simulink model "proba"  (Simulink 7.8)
settings: Solver=ode45  StartTime=0.0  StopTime=0.06  RelTol=1e-3
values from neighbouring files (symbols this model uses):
  alfa = 5*10e-3/6    (= 0.00833333333333)    [parametri.m]
  C = 3*C    (= 0.0039788735773)    [parametri.m]
  L = 7.64e-3    (= 0.00764)    [parametri.m]
  Lm = (9.3e-3)/W    (= 2.96028194151e-05)    [parametri.m]
  Rl = 1    [parametri.m]
  Rm = 1.6e-3    (= 0.0016)    [parametri.m]
libraries: powerlib x15, powerlib_extras x1

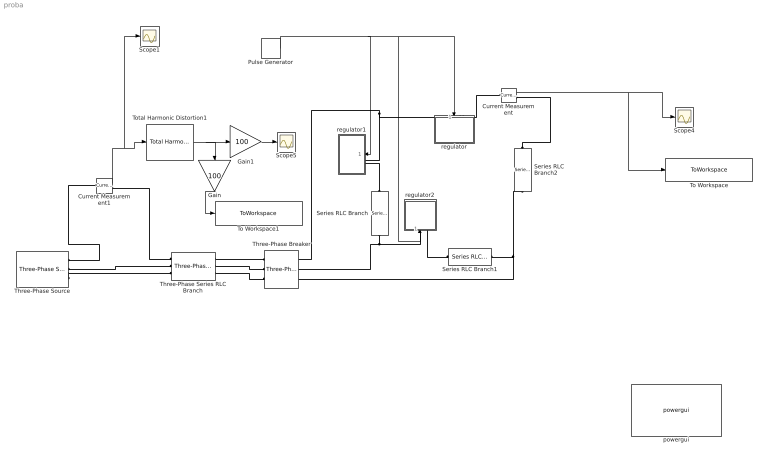
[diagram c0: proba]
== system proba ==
  Current Measurement : powerlib/Measurements/Current Measurement  PhasorSimulation=off  OutputType=Complex  PSBequivalent=0
  Current Measurement1 : powerlib/Measurements/Current Measurement  PhasorSimulation=off  OutputType=Complex  PSBequivalent=0
  Gain : Gain  Gain=100
  Gain1 : Gain  Gain=100  OutMin=0
  Pulse Generator : DiscretePulseGenerator  PulseType=Time based  Period=10e-3  PulseWidth=5  PhaseDelay=alfa
  Scope1 : Scope
  Scope4 : Scope
  Scope5 : Scope
  Series RLC Branch : powerlib/Elements/Series RLC Branch  LConnTagsString=__new0  RConnTagsString=__new0  BranchType=RL  Resistance=Rl  Inductance=L  SetiL0=off  InitialCurrent=0  Capacitance=C/3  Setx0=off  InitialVoltage=0  Measurements=None
  Series RLC Branch1 : powerlib/Elements/Series RLC Branch  LConnTagsString=__new0  RConnTagsString=__new0  BranchType=RL  Resistance=Rl  Inductance=L  SetiL0=off  InitialCurrent=0  Capacitance=C/3  Setx0=off  InitialVoltage=0  Measurements=None
  Series RLC Branch2 : powerlib/Elements/Series RLC Branch  LConnTagsString=__new0  RConnTagsString=__new0  BranchType=RL  Resistance=Rl  Inductance=L  SetiL0=off  InitialCurrent=0  Capacitance=C/3  Setx0=off  InitialVoltage=0  Measurements=None
  Three-Phase Series RLC Branch : powerlib/Elements/Three-Phase Series RLC Branch  LConnTagsString=A|B|C  RConnTagsString=A|B|C  BranchType=RL  Resistance=Rm  Inductance=Lm  Capacitance=1e-6  Measurements=None
  Three-Phase Breaker : powerlib/Elements/Three-Phase Breaker  InitialState=open  SwitchA=on  SwitchB=on  SwitchC=on  SwitchTimes="[0/50  1000/50]"  External=off  BreakerResistance=0.001  SnubberResistance=1e6  SnubberCapacitance=inf  Measurements=None
  Three-Phase Source : powerlib/Electrical Sources/Three-Phase Source  Voltage=400  PhaseAngle=0  Frequency=50  InternalConnection=Yg  SpecifyImpedance=off  Resistance=0  Inductance=0  ShortCircuitLevel=100e6  BaseVoltage=400  XRratio=7  BusType=swing  Pref=0  Qref=0  Qmin=-inf  Qmax=inf
  To Workspace : ToWorkspace  VariableName=struja_regulatora  SampleTime=-1  SaveFormat=Structure With Time
  To Workspace1 : ToWorkspace  VariableName=THD  SampleTime=-1  SaveFormat=Structure With Time
  Total Harmonic Distortion1 : powerlib_extras/Measurements/Total Harmonic Distortion  f1=50
  powergui : powerlib/powergui  Priority=1  SimulationMode=Continuous  SolverType=Tustin  SampleTime=50e-6  frequency=60  SPID=on  DisableSnubberDevices=on  DisableRonSwitches=on  DisableVfSwitches=on  SwTol=0  Interpol=off  DisplayEquations=on  FunctionMessages=off  frequencyindice=50  Pbase=100e6  ErrMax=1e-4  Iterations=50  UnitsV=kV  UnitsW=MW  echomessages=off  HookPort=off  EnableUseOfTLC=off  x0status=blocks  RestoreLinks=warning  ResistiveCurrentMeasurement=off  Ylog=off  Xlog=on  ShowGrid=off  save=off  variable=ZData  ZoomFFT=off  StartTime=0.0  cycles=1  DisplayStyle=1  FreqAxis=off  MaxFrequency=1000  frequencyindicesteady=1  RmsSteady=2  display=off  methode=off
  regulator : Subsystem
  regulator1 : Subsystem
  regulator2 : Subsystem
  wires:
  Current Measurement/1 -> Scope4/1, To Workspace/1
  Pulse Generator/1 -> regulator1/1(impulsi), regulator/1(impulsi), regulator2/1(impulsi)
  Current Measurement1/1 -> Total Harmonic Distortion1/1, Scope1/1
  Total Harmonic Distortion1/1 -> Gain/1, Gain1/1
  Gain/1 -> To Workspace1/1
  Gain1/1 -> Scope5/1
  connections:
  Three-Phase Source/RConn2 -- Three-Phase Series RLC Branch/LConn2
  Three-Phase Source/RConn3 -- Three-Phase Series RLC Branch/LConn3
  regulator1/LConn1 -- regulator/LConn1 -- Three-Phase Breaker/RConn1
  Series RLC Branch/RConn1 -- regulator2/LConn1 -- Three-Phase Breaker/RConn2
  Series RLC Branch1/RConn1 -- Series RLC Branch2/RConn1 -- Three-Phase Breaker/RConn3
  Current Measurement/LConn1 -- regulator/LConn2
  Series RLC Branch2/LConn1 -- Current Measurement/RConn1
  regulator2/LConn2 -- Series RLC Branch1/LConn1
  Series RLC Branch/LConn1 -- regulator1/LConn2
  Current Measurement1/LConn1 -- Three-Phase Source/RConn1
  Current Measurement1/RConn1 -- Three-Phase Series RLC Branch/LConn1
  Three-Phase Breaker/LConn1 -- Three-Phase Series RLC Branch/RConn1
  Three-Phase Breaker/LConn2 -- Three-Phase Series RLC Branch/RConn2
  Three-Phase Breaker/LConn3 -- Three-Phase Series RLC Branch/RConn3

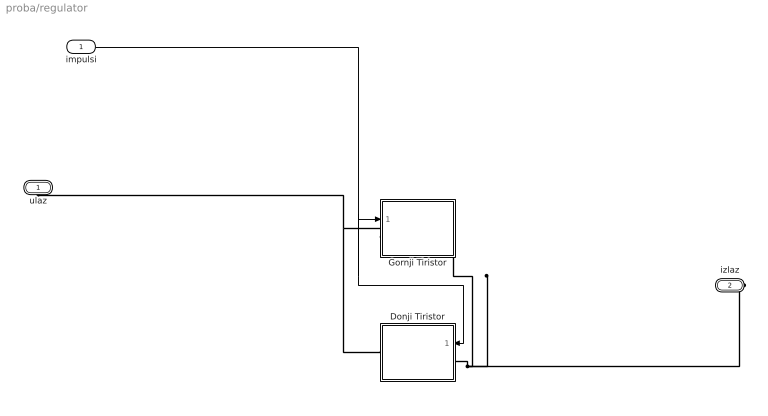
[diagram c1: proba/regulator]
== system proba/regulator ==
  impulsi : Inport
  Donji Tiristor : Subsystem
  Gornji Tiristor : Subsystem
  ulaz : PMIOPort  Port=1  Side=Left
  izlaz : PMIOPort  Port=2  Side=Left
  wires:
  impulsi/1 -> Gornji Tiristor/1(impulsi), Donji Tiristor/1(impulsi)
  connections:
  Donji Tiristor/LConn1 -- izlaz/RConn1 -- Gornji Tiristor/RConn1
  Donji Tiristor/RConn1 -- ulaz/RConn1 -- Gornji Tiristor/LConn1

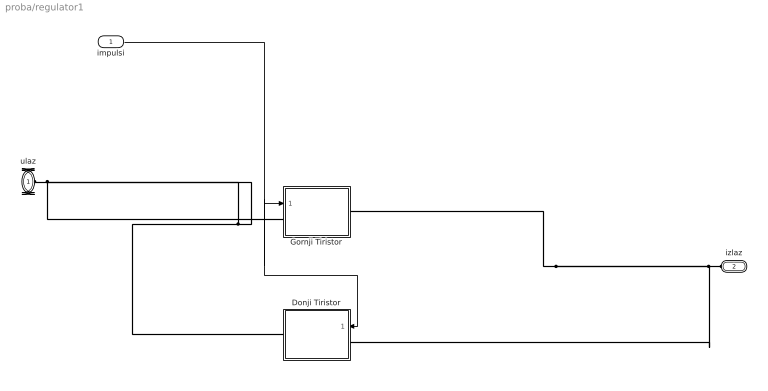
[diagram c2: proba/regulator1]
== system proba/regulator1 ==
  impulsi : Inport
  Donji Tiristor : Subsystem
  Gornji Tiristor : Subsystem
  ulaz : PMIOPort  Port=1  Side=Left
  izlaz : PMIOPort  Port=2  Side=Left
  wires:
  impulsi/1 -> Gornji Tiristor/1(impulsi), Donji Tiristor/1(impulsi)
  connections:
  izlaz/RConn1 -- Donji Tiristor/LConn1 -- Gornji Tiristor/RConn1
  ulaz/RConn1 -- Donji Tiristor/RConn1 -- Gornji Tiristor/LConn1

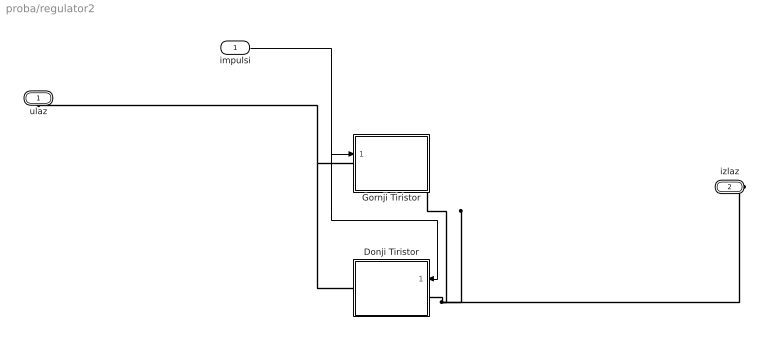
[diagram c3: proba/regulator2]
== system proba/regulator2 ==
  impulsi : Inport
  Donji Tiristor : Subsystem
  Gornji Tiristor : Subsystem
  ulaz : PMIOPort  Port=1  Side=Left
  izlaz : PMIOPort  Port=2  Side=Left
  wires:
  impulsi/1 -> Gornji Tiristor/1(impulsi), Donji Tiristor/1(impulsi)
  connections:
  Donji Tiristor/LConn1 -- izlaz/RConn1 -- Gornji Tiristor/RConn1
  Donji Tiristor/RConn1 -- ulaz/RConn1 -- Gornji Tiristor/LConn1

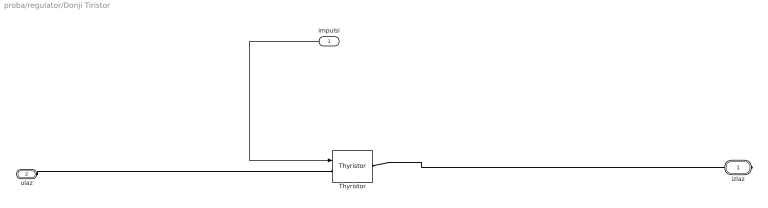
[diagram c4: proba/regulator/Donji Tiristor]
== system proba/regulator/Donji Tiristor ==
  impulsi : Inport
  Thyristor : powerlib/Power Electronics/Thyristor  Ron=1e-3  Lon=0  Vf=0.8  IC=0  Rs=20  Cs=4e-6  Measurements=off
  izlaz : PMIOPort  Port=1  Side=Right
  ulaz : PMIOPort  Port=2  Side=Left
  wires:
  impulsi/1 -> Thyristor/1
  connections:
  Thyristor/RConn1 -- izlaz/RConn1
  ulaz/RConn1 -- Thyristor/LConn1

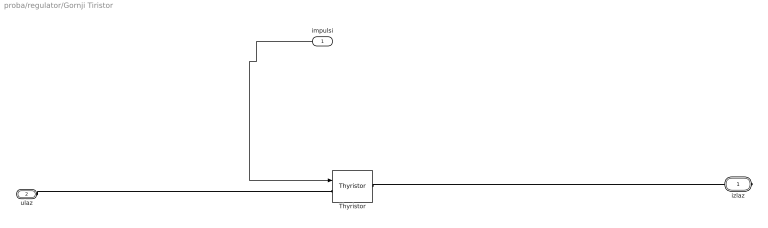
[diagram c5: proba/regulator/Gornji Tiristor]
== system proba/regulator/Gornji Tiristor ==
  impulsi : Inport
  Thyristor : powerlib/Power Electronics/Thyristor  Ron=1e-3  Lon=0  Vf=0.8  IC=0  Rs=20  Cs=4e-6  Measurements=off
  izlaz : PMIOPort  Port=1  Side=Right
  ulaz : PMIOPort  Port=2  Side=Left
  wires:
  impulsi/1 -> Thyristor/1
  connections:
  Thyristor/RConn1 -- izlaz/RConn1
  ulaz/RConn1 -- Thyristor/LConn1

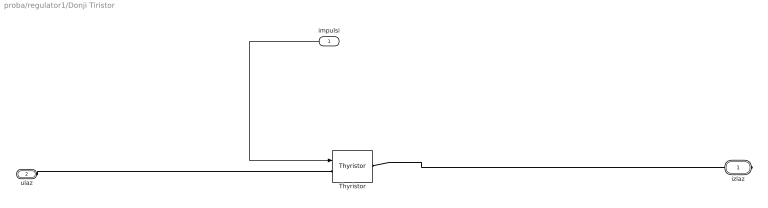
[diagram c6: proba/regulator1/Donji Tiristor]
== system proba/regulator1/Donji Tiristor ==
  impulsi : Inport
  Thyristor : powerlib/Power Electronics/Thyristor  Ron=1e-3  Lon=0  Vf=0.8  IC=0  Rs=20  Cs=4e-6  Measurements=off
  izlaz : PMIOPort  Port=1  Side=Right
  ulaz : PMIOPort  Port=2  Side=Left
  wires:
  impulsi/1 -> Thyristor/1
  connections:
  Thyristor/RConn1 -- izlaz/RConn1
  ulaz/RConn1 -- Thyristor/LConn1

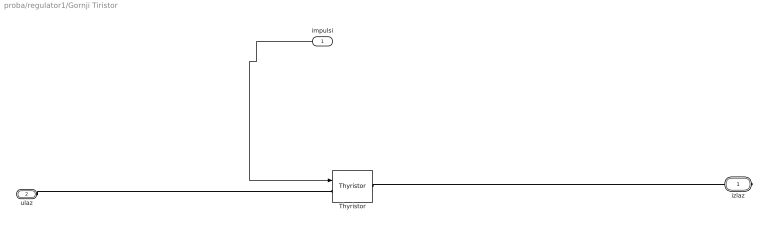
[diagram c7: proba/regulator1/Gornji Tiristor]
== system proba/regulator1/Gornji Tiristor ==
  impulsi : Inport
  Thyristor : powerlib/Power Electronics/Thyristor  Ron=1e-3  Lon=0  Vf=0.8  IC=0  Rs=20  Cs=4e-6  Measurements=off
  izlaz : PMIOPort  Port=1  Side=Right
  ulaz : PMIOPort  Port=2  Side=Left
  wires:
  impulsi/1 -> Thyristor/1
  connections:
  Thyristor/RConn1 -- izlaz/RConn1
  ulaz/RConn1 -- Thyristor/LConn1

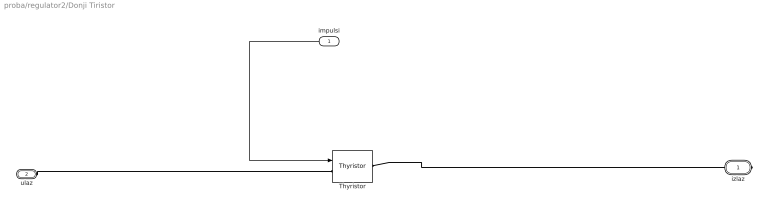
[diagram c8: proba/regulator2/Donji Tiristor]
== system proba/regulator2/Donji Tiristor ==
  impulsi : Inport
  Thyristor : powerlib/Power Electronics/Thyristor  Ron=1e-3  Lon=0  Vf=0.8  IC=0  Rs=20  Cs=4e-6  Measurements=off
  izlaz : PMIOPort  Port=1  Side=Right
  ulaz : PMIOPort  Port=2  Side=Left
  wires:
  impulsi/1 -> Thyristor/1
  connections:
  Thyristor/RConn1 -- izlaz/RConn1
  ulaz/RConn1 -- Thyristor/LConn1

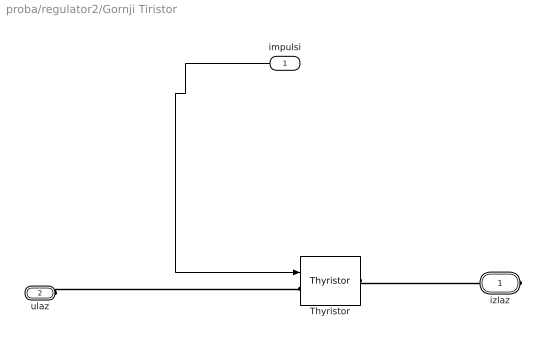
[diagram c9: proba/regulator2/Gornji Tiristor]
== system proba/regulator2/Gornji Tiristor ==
  impulsi : Inport
  Thyristor : powerlib/Power Electronics/Thyristor  Ron=1e-3  Lon=0  Vf=0.8  IC=0  Rs=20  Cs=4e-6  Measurements=off
  izlaz : PMIOPort  Port=1  Side=Right
  ulaz : PMIOPort  Port=2  Side=Left
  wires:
  impulsi/1 -> Thyristor/1
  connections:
  Thyristor/RConn1 -- izlaz/RConn1
  ulaz/RConn1 -- Thyristor/LConn1
